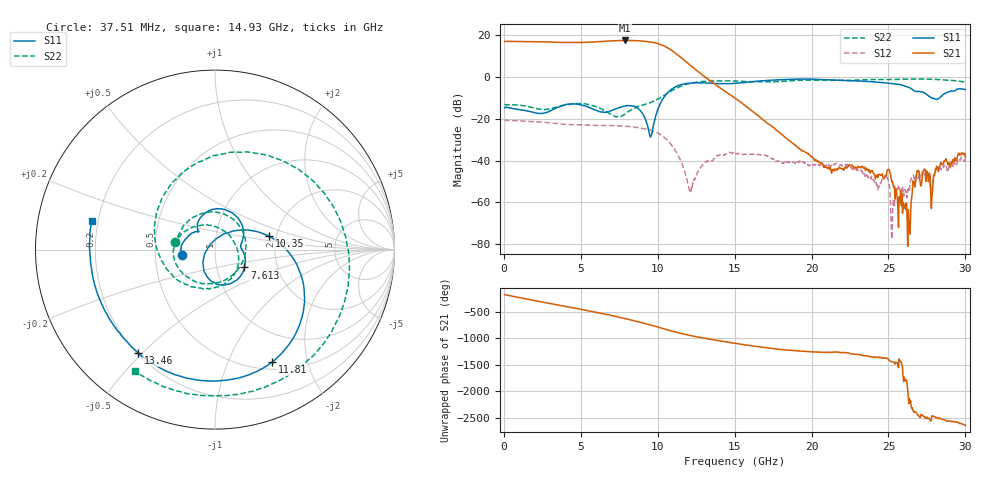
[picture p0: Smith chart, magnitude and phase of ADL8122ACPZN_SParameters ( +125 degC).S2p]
! "Analog Devices, Inc."
! Device:	ADL8122ACPZN
! Description:	"10 kHz to 10 GHz, Wideband, Low Noise Amplifier"
! Conditions:	Vdd = 5.0 V
!		IDQ = 95 mA
!		Pin = -25 dBm
!		Operating Temperature = +25 C (at package bottom)
! Product validation unit SN1 soldered down to Evaluation Board as shown on ADL8122-EVALZ User Guide. Board loss de-embedded from S21 magnitude.  All other RF measurements reference to RF coaxial connector.
! Frequency (GHz)	S11_Mag (dB)	S11_Phase (deg)	S21_Mag (dB)	S21_Phase (deg)	S12_Mag (dB)	S12_Phase (deg)	S22_Mag (dB)	S22_Phase (deg)
#  GHZ  S  DB  R 50
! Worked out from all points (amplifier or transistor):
!   800 points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, 37.51 MHz to 30 GHz, reference 50 ohm
!   highest |S21| = 17.6 dB at 7.875 GHz (marker M1)
!   |S21| within 3 dB of that: start of sweep to 10.5 GHz
!   unconditionally stable (mu >= 1): start of sweep to end of sweep
!   at 5.025 GHz: K = 1.20, MAG = 17.0 dB, |S12| = -22.9 dB
!   at 15.04 GHz: K = 17.59, MAG = -2.3 dB, |S12| = -36.4 dB
!   at 30 GHz: K = 1605.92, MAG = -33.4 dB, |S12| = -41.8 dB
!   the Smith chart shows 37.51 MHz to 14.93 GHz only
!   S11 on the Smith chart (normalised r, x): 37.51 MHz: 0.69, -0.04; 7.613 GHz: 1.36, -0.28; 10.35 GHz: 1.84, +0.30; 11.81 GHz: 0.59, -1.46; 13.46 GHz: 0.20, -0.48; 14.93 GHz: 0.17, +0.11
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0.03750899  -14.68 -170.2  17.11 -178.7  -20.67 1.3  -12.90 169.7
1.537508  -16.28 141.8  17.07 93.2  -21.13 -75.7  -14.04 64.7
2.212508  -17.30 132.8  17.00 55.2  -21.40 -109.0  -15.13 9.2
3.000008  -16.18 128.9  16.85 11.0  -21.89 -148.3  -15.11 -64.7
4.162508  -12.94 90.9  16.62 -51.3  -22.60 155.0  -13.16 -141.2
5.062508  -13.37 51.8  16.66 -100.2  -22.85 110.2  -12.66 -177.1
6.450007  -16.81 7.9  17.15 179.7  -23.05 36.5  -15.69 126.5
7.612507  -14.36 -31.2  17.59 105.5  -23.40 -29.4  -18.77 17.8
7.875006  -13.81 -45.3  17.61 87.9  -23.46 -45.1  -17.62 -10.2
8.400007  -13.83 -75.5  17.56 51.5  -23.86 -76.7  -15.09 -52.9
9.000007  -17.25 -116.1  17.32 7.9  -24.56 -113.4  -13.34 -91.9
9.487506  -28.03 165.3  16.91 -29.5  -25.30 -146.2  -12.18 -122.9
10.05001  -14.49 35.7  15.98 -75.6  -26.97 173.0  -10.28 -169.0
10.35001  -10.12 13.9  15.14 -100.9  -28.45 150.0  -9.02 162.6
10.95001  -5.46 -22.1  12.59 -150.5  -33.16 104.8  -6.27 104.5
11.81251  -3.06 -63.1  7.56 147.9  -46.85 33.8  -3.52 35.1
13.46251  -2.88 -126.8  -2.04 56.0  -39.64 164.6  -1.81 -59.2
14.925  -3.02 166.8  -9.51 -12.9  -36.37 97.0  -1.84 -123.2
15.0375  -2.94 161.2  -10.09 -18.2  -36.41 94.4  -1.85 -127.9
20.025  -0.93 13.3  -38.31 -175.6  -42.05 -60.9  -1.46 45.1
25.0125  -2.89 -121.1  -44.17 32.5  -50.28 69.6  -1.10 -106.1
30  -5.92 -111.6  -38.48 -125.4  -41.79 -127.5  -2.35 -165.6
